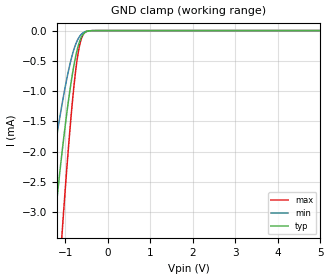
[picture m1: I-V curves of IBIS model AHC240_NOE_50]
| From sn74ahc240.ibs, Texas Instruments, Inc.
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[Model]   AHC240_NOE_50
Model_type  Input
Vinl=1.65
Vinh=3.85
| variable   typ   min   max
C_comp   0.59pF   0.51pF   0.67pF
[Temperature Range]   40   100   -40
| Ambient temperature   25   85   -40
[Voltage range]   5   4.5   5.5
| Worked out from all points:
|   GND clamp passes 1 mA (typ) near -0.90 V on its own axis
[GND Clamp]
| AHC240_NOE_50
|   Voltage   I(typ)   I(min)   I(max)
-5V       -42.63mA   -27.8mA    -54.13mA
-1.56V    -5.495mA   -3.489mA   -8.664mA
-1.51V    -5.091mA   -3.226mA   -8.077mA
-1.28V    -3.347mA   -2.09mA    -5.468mA
-1.08V    -2.016mA   -1.22mA    -3.363mA
-1.06V    -1.895mA   -1.141mA   -3.164mA
-900mV    -1.015mA   -576.4uA   -1.69mA
-770mV    -465.9uA   -248.7uA   -730.8uA
-670mV    -187.3uA   -100.6uA   -256.8uA
-620mV    -101.8uA   -57.6uA    -126.1uA
-550mV    -35.83uA   -22.61uA   -37.11uA
5V        15.07nA    1.006nA    138.2nA
